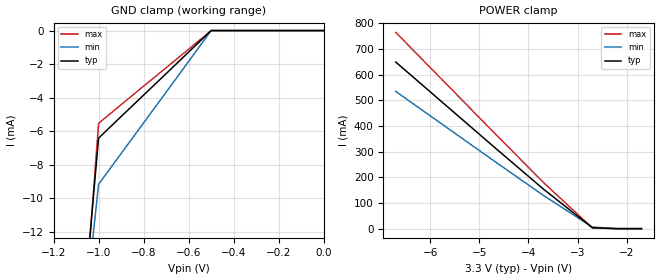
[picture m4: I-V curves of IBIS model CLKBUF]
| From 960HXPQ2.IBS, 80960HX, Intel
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|This is the model for the buffer CLKBUF.
[Model] CLKBUF
Model_type Input
Polarity Non-Inverting
Enable Active-High
|Signals  CLKIN
Vinl = 0.8V
Vinh = 2.0V
|variable   typ   min   max
C_comp   2.1pf	1.9pf	2.3pf
|variable   typ   min   max
[Voltage range]   3.3V   3.0V   3.6V
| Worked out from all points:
|   GND clamp passes 1 mA (typ) near -0.58 V on its own axis
|   POWER clamp passes 1 mA (typ) near -2.33 V on its own axis
[GND_Clamp]
|Voltage   I(typ)   I(min)   I(max)
-5V       -653.7mA   -539.2mA   -769.6mA
-2V       -159.1mA   -134.8mA   -185.5mA
-1V       -6.42mA    -9.176mA   -5.534mA
-900mV    -5.13mA    -7.339mA   -4.425mA
-800mV    -3.85mA    -5.51mA    -3.316mA
-700mV    -2.57mA    -3.674mA   -2.218mA
-600mV    -1.28mA    -1.837mA   -1.109mA
-500mV    0A         0A         0A
-400mV    0A         0A         0A
0V        0A         0A         0A
|Note that the voltages in the Power_clamp data table are Vcc relative
|which means they are referenced to Vcc.  The voltages in the table are
|derived from the following equation:
|Vtable = Vcc - Voutput
|0V in the table is actually 3.3V with respect to ground and 0V above Vcc.
[POWER_Clamp]
|Voltage   I(typ)   I(min)   I(max)
-6.7V     648.4mA    534.1mA    763.9mA
-4.7V     318mA      263.5mA    373.7mA
-3.7V     154.7mA    130.1mA    180.7mA
-2.7V     3.83mA     6.232mA    2.997mA
-2.6V     3.06mA     4.986mA    2.407mA
-2.5V     2.23mA     3.739mA    1.805mA
-2.4V     1.53mA     2.46mA     1.18mA
-2.3V     770uA      1.246mA    601.8uA
-2.2V     0A         0A         0A
-1.7V     0A         0A         0A
